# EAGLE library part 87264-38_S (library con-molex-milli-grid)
RECEPTACAL
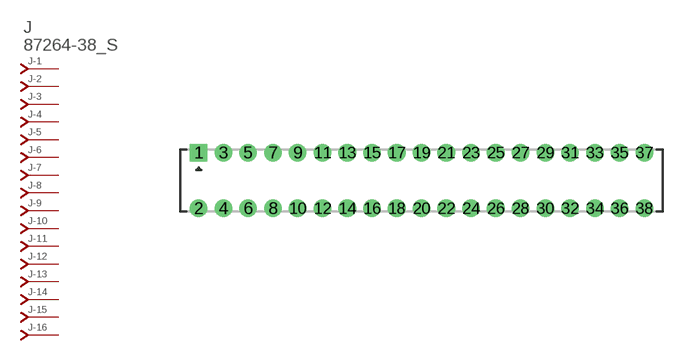
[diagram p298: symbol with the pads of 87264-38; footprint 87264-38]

Designator prefix J; gates -1=J-NV -2=J-N -3=J-N -4=J-N -5=J-N -6=J-N -7=J-N -8=J-N -9=J-N -10=J-N -11=J-N -12=J-N -13=J-N -14=J-N -15=J-N -16=J-N -17=J-N -18=J-N -19=J-N -20=J-N -21=J-N -22=J-N -23=J-N -24=J-N -25=J-N -26=J-N -27=J-N -28=J-N -29=J-N -30=J-N -31=J-N -32=J-N -33=J-N -34=J-N -35=J-N -36=J-N -37=J-N -38=J-N

## 87264-38_S  [87264-38]
1  -1:J  pas
2  -2:J  pas
3  -3:J  pas
4  -4:J  pas
5  -5:J  pas
6  -6:J  pas
7  -7:J  pas
8  -8:J  pas
9  -9:J  pas
10  -10:J  pas
11  -11:J  pas
12  -12:J  pas
13  -13:J  pas
14  -14:J  pas
15  -15:J  pas
16  -16:J  pas
17  -17:J  pas
18  -18:J  pas
19  -19:J  pas
20  -20:J  pas
21  -21:J  pas
22  -22:J  pas
23  -23:J  pas
24  -24:J  pas
25  -25:J  pas
26  -26:J  pas
27  -27:J  pas
28  -28:J  pas
29  -29:J  pas
30  -30:J  pas
31  -31:J  pas
32  -32:J  pas
33  -33:J  pas
34  -34:J  pas
35  -35:J  pas
36  -36:J  pas
37  -37:J  pas
38  -38:J  pas

## Footprint 87264-38 (pad centres in mm)
RECEPTACAL Dual Row, Side Entry
drill 0.914 square: 1 -18,2.25
drill 0.914: 2 -18,-2.25; 3 -16,2.25; 4 -16,-2.25; 5 -14,2.25; 6 -14,-2.25; 7 -12,2.25; 8 -12,-2.25; 9 -10,2.25; 10 -10,-2.25; 11 -8,2.25; 12 -8,-2.25; 13 -6,2.25; 14 -6,-2.25; 15 -4,2.25; 16 -4,-2.25; 17 -2,2.25; 18 -2,-2.25; 19 0,2.25; 20 0,-2.25; 21 2,2.25; 22 2,-2.25; 23 4,2.25; 24 4,-2.25; 25 6,2.25; 26 6,-2.25; 27 8,2.25; 28 8,-2.25; 29 10,2.25; 30 10,-2.25; 31 12,2.25; 32 12,-2.25; 33 14,2.25; 34 14,-2.25; 35 16,2.25; 36 16,-2.25; 37 18,2.25; 38 18,-2.25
